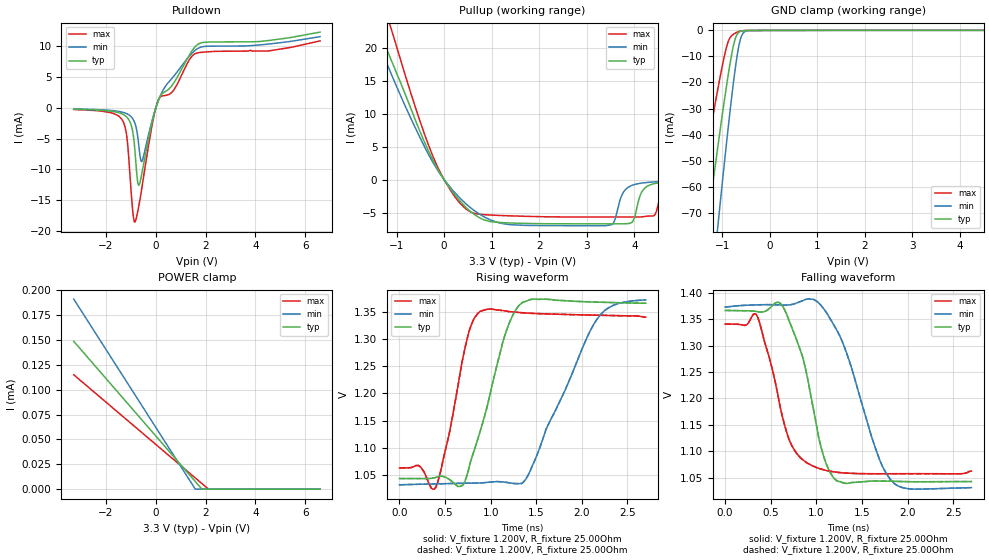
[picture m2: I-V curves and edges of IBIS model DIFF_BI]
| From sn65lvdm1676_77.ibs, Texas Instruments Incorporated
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|   Driver Output/Receiver Input Model
[Model]   DIFF_BI
Model_type   I/O
| Signals   A1Y,A1Z,A2Y,A2Z,A3Y,A3Z,A4Y,A4Z,B1Y,B1Z,B2Y,B2Z,B3Y,B3Z,B4Y,B4Z,
|   C1Y,C1Z,C2Y,C2Z,C3Y,C3Z,C4Y,C4Z,D1Y,D1Z,D2Y,D2Z,D3Y,D3Z,D4Y,D4Z
Vinl  = 1.0V
Vinh  = 1.4V
Vmeas = 1.2V   |Reference voltage for timing measurements
Cref  = 10pF   |Timing specification test load capacitance value
Rref  = 50   |Note: 50 Ohm load; single ended configuration
Vref  = 1.18V   |Timing specification test load voltage
| variable   typ   min   max
|C_comp avg
|C_comp   4.116pF   3.789pF   3.708pF
|C_comp in RCV mode
C_comp   3.064pF   3.159pF   2.939pF
|C_comp in DRV mode
|C_comp   4.592pF   4.419pF   4.744pF
|   typ   min   max
| Junction Temperature (Ambient temp is 25C typ, 85C min, 0C max)
[Temperature Range]   40.0   100   -40
[Voltage range]   3.3V   3.0V   3.6V
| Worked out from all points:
|   slope of the pulldown table from 0 to 0.495 V, typ, clamps not added: 168 ohm
|   slope of the pullup table from 0 to 0.495 V, typ, clamps not added: 111 ohm
|   GND clamp passes 1 mA (typ) near -0.67 V on its own axis
|   falling waveform, V_fixture 1.200V, R_fixture 25.00Ohm: 20-80 % time 249ps typ, 370ps min, 241ps max; typ from 1.37 V to 1.04 V
|   rising waveform, V_fixture 1.200V, R_fixture 25.00Ohm: 20-80 % time 302ps typ, 522ps min, 185ps max; typ from 1.04 V to 1.37 V
|   rising waveform, V_fixture 1.200V, R_fixture 25.00Ohm: 20-80 % time 302ps typ, 522ps min, 185ps max; typ from 1.04 V to 1.37 V
|   falling waveform, V_fixture 1.200V, R_fixture 25.00Ohm: 20-80 % time 249ps typ, 370ps min, 241ps max; typ from 1.37 V to 1.04 V
[Pulldown]
|   Voltage   I(typ)   I(min)   I(max)
-3.3V     -225uA     -190.1uA   -272.9uA
-1.315V   -1.085mA   -747.1uA   -2.234mA
-1.166V   -1.52mA    -964.3uA   -4.663mA
-942.9mV  -3.564mA   -1.688mA   -16.08mA
-843.6mV  -6.747mA   -2.47mA    -18.56mA
-719.5mV  -12.26mA   -4.889mA   -16.68mA
-570.7mV  -10.86mA   -8.729mA   -13.25mA
-198.5mV  -3.213mA   -2.831mA   -3.903mA
74.44mV   897.9uA    867.6uA    989.4uA
719.5mV   4.02mA     5.117mA    2.872mA
1.464V    9.3mA      8.893mA    8.423mA
6.6V      12.28mA    11.54mA    10.85mA
[GND Clamp]
|   Voltage   I(typ)   I(min)   I(max)
-3.3V     -362.3mA   -502.6mA   -261.1mA
-1.638V   -119.6mA   -175.9mA   -78.76mA
-1.588V   -112.6mA   -166.5mA   -73.48mA
-1.315V   -74.51mA   -115.4mA   -44.82mA
-1.092V   -44.28mA   -74.69mA   -22.27mA
-893.2mV  -19.09mA   -40.17mA   -5.252mA
-769.2mV  -6.124mA   -20.5mA    -1.547mA
-694.7mV  -1.731mA   -10.47mA   -772.9uA
-645.1mV  -660.7uA   -5.353mA   -436.2uA
-595.5mV  -267uA     -2.15mA    -219.2uA
-446.6mV  -60.63uA   -116.8uA   -45.67uA
6.6V      0A         0A         0A
[Pullup]
|   Voltage   I(typ)   I(min)   I(max)
-3.3V     63.08mA    58.38mA    72.42mA
-1.563V   26.35mA    24.09mA    32.69mA
-1.166V   19.13mA    17.01mA    24.14mA
-124.1mV  1.478mA    1.314mA    1.737mA
347.4mV   -3.344mA   -2.887mA   -3.657mA
843.6mV   -6.104mA   -5.65mA    -5.298mA
3.399V    -6.693mA   -6.97mA    -5.654mA
3.995V    -5.935mA   -735.1uA   -5.657mA
4.144V    -2.043mA   -509uA     -5.639mA
4.392V    -634.2uA   -332.4uA   -5.497mA
4.764V    -293.6uA   -216.4uA   -585.9uA
6.6V      -76.6uA    -76.7uA    -65.6uA
[POWER Clamp]
|   Voltage   I(typ)   I(min)   I(max)
-3.3V     148.7uA    191.2uA    115.1uA
1.588V    7.64uA     0A         11.24uA
1.861V    0A         0A         5.448uA
2.134V    0A         0A         0A
6.6V      0A         0A         0A
[Ramp]
R_load = 25.00Ohm
|   typ   min   max
dV/dt_r   194.332mV/301.988ps 204.991mV/521.266ps 167.026mV/184.577ps
dV/dt_f   194.332mV/248.917ps 204.991mV/369.417ps 167.026mV/240.643ps
[Falling Waveform]
V_fixture = 1.200V
V_fixture_min = 1.200V
V_fixture_max = 1.200V
R_fixture = 25.00Ohm
|   Time   V(typ)   V(min)   V(max)
0s        1.367V     1.373V     1.341V
348ps     1.364V     1.377V     1.357V
627ps     1.375V     1.377V     1.166V
825ps     1.291V     1.383V     1.088V
1.052ns   1.107V     1.376V     1.066V
1.218ns   1.045V     1.331V     1.061V
1.384ns   1.041V     1.259V     1.058V
1.652ns   1.044V     1.104V     1.058V
1.816ns   1.043V     1.046V     1.058V
2.7ns     1.043V     1.031V     1.062V
[Rising Waveform]
V_fixture = 1.200V
V_fixture_min = 1.200V
V_fixture_max = 1.200V
R_fixture = 25.00Ohm
|   Time   V(typ)   V(min)   V(max)
0s        1.043V     1.031V     1.062V
213ps     1.043V     1.032V     1.067V
399ps     1.045V     1.033V     1.027V
540ps     1.042V     1.034V     1.121V
699ps     1.032V     1.034V     1.268V
888ps     1.132V     1.035V     1.352V
1.153ns   1.306V     1.036V     1.353V
1.341ns   1.367V     1.034V     1.349V
2.159ns   1.369V     1.335V     1.345V
2.7ns     1.367V     1.373V     1.341V
[Rising Waveform]
V_fixture = 1.200V
V_fixture_min = 1.200V
V_fixture_max = 1.200V
R_fixture = 25.00Ohm
|   Time   V(typ)   V(min)   V(max)
0s        1.043V     1.031V     1.062V
213ps     1.043V     1.032V     1.067V
399ps     1.045V     1.033V     1.027V
540ps     1.042V     1.034V     1.121V
699ps     1.032V     1.034V     1.268V
889ps     1.132V     1.035V     1.352V
1.154ns   1.306V     1.036V     1.353V
1.341ns   1.367V     1.034V     1.349V
2.159ns   1.369V     1.335V     1.345V
2.7ns     1.367V     1.373V     1.341V
[Falling Waveform]
V_fixture = 1.200V
V_fixture_min = 1.200V
V_fixture_max = 1.200V
R_fixture = 25.00Ohm
|   Time   V(typ)   V(min)   V(max)
0s        1.367V     1.373V     1.341V
348ps     1.364V     1.377V     1.357V
627ps     1.375V     1.377V     1.166V
710ps     1.343V     1.377V     1.119V
826ps     1.291V     1.383V     1.088V
1.052ns   1.107V     1.376V     1.066V
1.218ns   1.045V     1.331V     1.061V
1.652ns   1.044V     1.104V     1.058V
1.816ns   1.043V     1.046V     1.058V
2.7ns     1.043V     1.031V     1.062V
